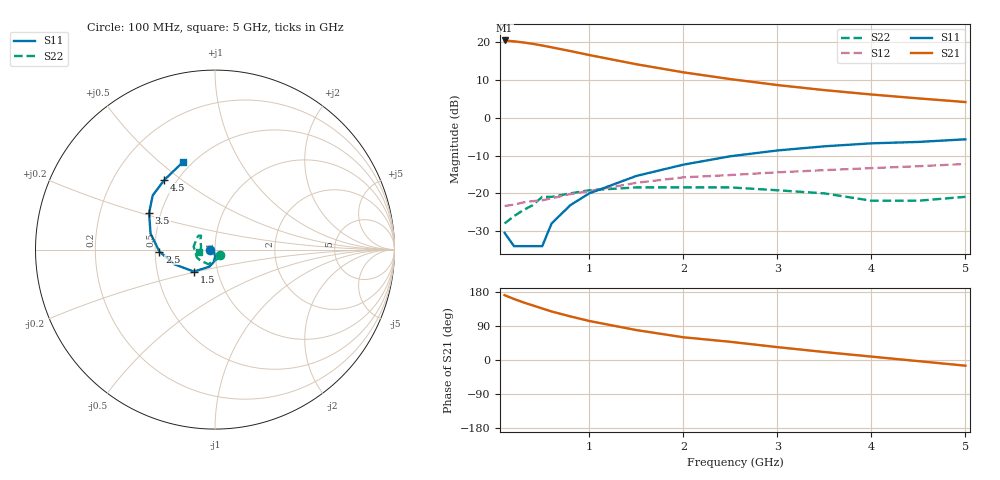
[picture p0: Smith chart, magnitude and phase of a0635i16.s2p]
!  MSA-0635 S AND NOISE PARAMETERS
!  Id=16mA  LAST UPDATED 07-22-92
# ghz s ma r 50
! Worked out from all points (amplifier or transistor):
!   16 points, 100 MHz to 5 GHz, reference 50 ohm
!   highest |S21| = 20.5 dB at 100 MHz (marker M1)
!   |S21| within 3 dB of that: start of sweep to 835.6 MHz
!   unconditionally stable (mu >= 1): start of sweep to end of sweep
!   at 300 MHz: K = 1.04, MAG = 20.0 dB, |S12| = -22.4 dB
!   at 1.5 GHz: K = 1.02, MAG = 14.8 dB, |S12| = -17.2 dB
!   at 5 GHz: K = 1.08, MAG = 6.4 dB, |S12| = -12.2 dB
!   lowest NFmin = 2.70 dB at 100 MHz
!   S11 on the Smith chart (normalised r, x): 100 MHz: 0.94, -0.00; 1.5 GHz: 0.77, -0.19; 2.5 GHz: 0.53, -0.01; 3.5 GHz: 0.43, +0.21; 4.5 GHz: 0.43, +0.43; 5 GHz: 0.45, +0.60
0.1  0.03 -178.0  10.59 171.0  0.068 5.0  0.04 -44.0
0.2  0.02 -177.0  10.31 161.0  0.071 8.0  0.05 -68.0
0.3  0.02 -164.0  9.96 152.0  0.076 14.0  0.06 -87.0
0.4  0.02 -116.0  9.55 144.0  0.079 19.0  0.07 -104.0
0.5  0.02 -100.0  9.08 136.0  0.081 21.0  0.09 -114.0
0.6  0.04 -89.0  8.59 128.0  0.086 24.0  0.09 -123.0
0.8  0.07 -96.0  7.66 115.0  0.098 29.0  0.1 -140.0
1  0.1 -108.0  6.79 103.0  0.107 31.0  0.11 -156.0
1.5  0.17 -134.0  5.13 79.0  0.138 30.0  0.12 172.0
2  0.24 -160.0  4.01 60.0  0.163 26.0  0.12 148.0
2.5  0.31 -178.0  3.26 48.0  0.175 27.0  0.12 140.0
3  0.37 166.0  2.72 34.0  0.19 24.0  0.11 135.0
3.5  0.42 151.0  2.33 21.0  0.203 19.0  0.1 144.0
4  0.46 139.0  2.04 9.0  0.216 16.0  0.08 167.0
4.5  0.48 126.0  1.81 -3.0  0.229 12.0  0.08 -173.0
5  0.52 110.0  1.62 -15.0  0.245 8.0  0.09 -173.0
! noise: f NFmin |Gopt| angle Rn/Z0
0.1  2.7  0.12  4  0.41
0.5  2.8  0.1  19  0.4
1  3  0.08  44  0.38
2  3.3  0.06  167  0.35
